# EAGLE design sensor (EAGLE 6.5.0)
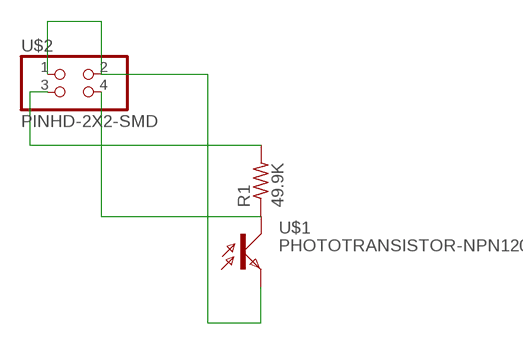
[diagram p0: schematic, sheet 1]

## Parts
R1  49.9K  RES-US1206FAB  [R1206FAB]
U$1  PHOTOTRANSISTOR-NPN1206  [OP1206]
U$2  PINHD-2X2-SMD  [2X02SMD]

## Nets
N$1: R1.1 U$1.COLLECTOR(C) U$2.4
N$2: U$1.EMITTER(E) U$2.1 U$2.2
N$5: R1.2 U$2.3

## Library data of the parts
R1 = fab:RES-US: Resistor (US Symbol)
U$1 = fab:PHOTOTRANSISTOR-NPN
U$2 = fab:PINHD-2X2-SMD

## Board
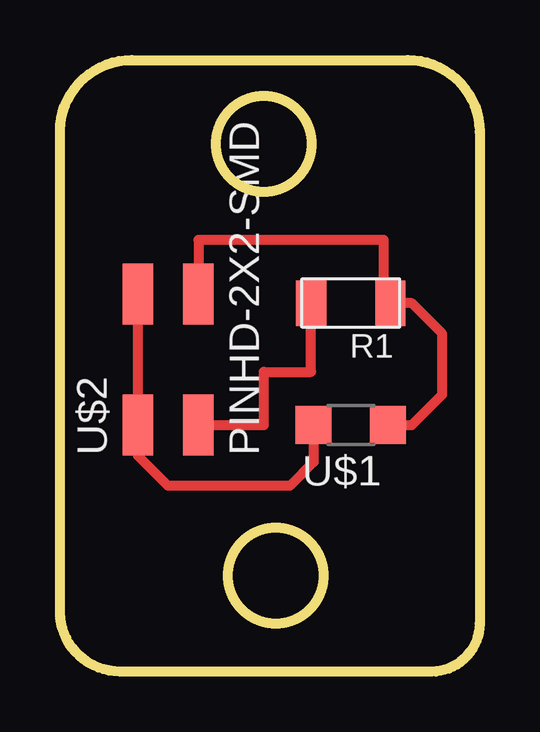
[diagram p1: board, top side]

Size 17.5 x 25.5 mm. Coordinates in mm from the lower left corner, seen from the top.
Outline: 3,25.5 14.5,25.5 arc-90 17.5,22.5 17.5,2 arc-90 15.5,0 2.5,0 arc-90 0,2.5 0,22.5 arc-90 3,25.5
Outline: circle at 9,4 radius 2
Outline: circle at 8.5,22 radius 2
Copper layers (1*16): Top 0.035mm / dielectric 1.5mm / Bottom 0.035mm
Design rules "default": minimum track width 10mil, minimum drill 24mil, track to track 8mil, track to pad 8mil, pad to pad 8mil, via to via 8mil, smd to smd 8mil, copper to edge 40mil, drill to drill 8mil, minimum pad ring 10mil, minimum via ring 8mil, stop-mask expansion 4mil, vias tented up to drill 0mil, thermal gap 10mil

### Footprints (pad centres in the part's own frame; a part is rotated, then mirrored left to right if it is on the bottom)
R1206FAB = smd 1.27 x 1.905: 1 -1.651,0; 2 1.651,0
OP1206 = smd 1.5 x 1.6: COLLECTOR -1.55,0; EMITTER 1.55,0
2X02SMD = smd 2.54 x 1.27: 1 -2.54,1.27; 2 2.92,1.27; 3 -2.54,-1.27; 4 2.92,-1.27

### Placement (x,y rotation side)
R1  12.13,15.36 180 top
U$1  12.13,10.28 180 top
U$2  4.51,12.82 90 top

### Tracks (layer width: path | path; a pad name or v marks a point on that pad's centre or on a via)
N$1
  Top 0.406: U$1.COLLECTOR 14.67,10.28 15.94,11.55 15.94,14.09 14.67,15.36 R1.1 13.5,15.36 13.5,18 5.78,18 U$2.4
N$2
  Top 0.406: U$1.EMITTER 10.58,8.73 9.59,7.74 4.51,7.74 3.24,9.01 U$2.1 U$2.2
N$5
  Top 0.406: U$2.3 8.5,10.28 8.5,12.5 10.48,12.5 R1.2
